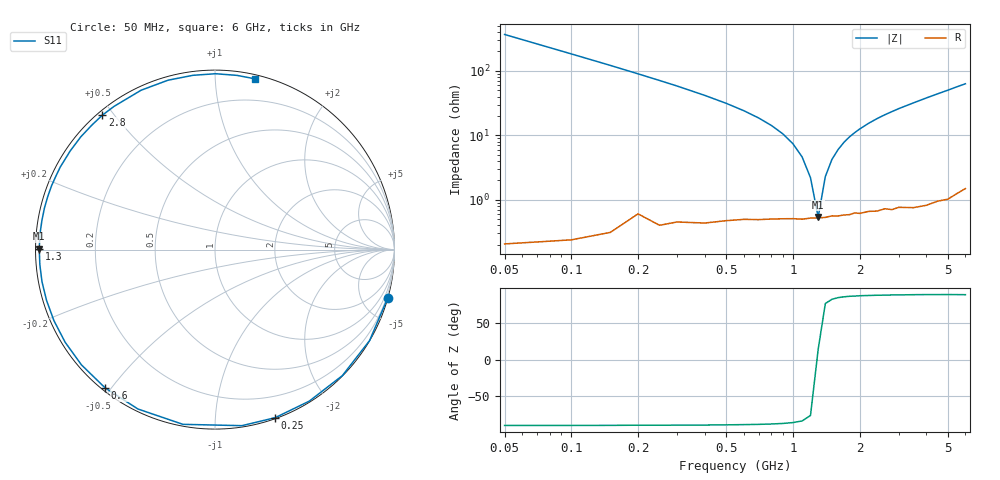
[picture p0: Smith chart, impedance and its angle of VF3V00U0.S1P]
! Infineon Technologies  Discrete & RF Semiconductors
! BBY 58-03
! Si Tuning Diode in SOD323
! VR = 3 V
! S-Parameters:  June  1999
# GHz  S  MA  R  50
!  f  S11
! GHz  MAG  ANG
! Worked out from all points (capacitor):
!   34 points, 50 MHz to 6 GHz, reference 50 ohm
!   read as one part to ground: C = 8.63 pF near 50 MHz
!   lowest |Z| = 539 mohm at 1.3 GHz (marker M1)
!   series resonance near 1.294 GHz, so ESL is about 1.8 nH
!   S11 on the Smith chart (normalised r, x): 50 MHz: 0.00, -7.35; 250 MHz: 0.01, -1.42; 600 MHz: 0.01, -0.48; 1.3 GHz: 0.01, +0.00; 2.8 GHz: 0.01, +0.47; 6 GHz: 0.03, +1.26
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0.05  0.9999 -15.5
0.1  0.9993 -30.5
0.15  0.9982 -44.7
0.2  0.9943 -58.1
0.25  0.9947 -70.3
0.3  0.9924 -81.3
0.4  0.9898 -100.4
0.5  0.9865 -115.8
0.6  0.984 -128.5
0.7  0.9829 -139.2
0.8  0.9816 -148.3
0.9  0.9808 -156.2
1  0.9803 -163.2
1.1  0.9804 -169.5
1.3  0.9793 179.7
1.5  0.9779 170.4
1.6  0.9781 166.3
1.8  0.9776 158.6
2  0.9772 151.9
2.4  0.9767 140.0
2.8  0.9772 129.9
3  0.9762 125.2
3.5  0.9788 114.9
4  0.9794 105.5
4.5  0.9788 97.2
5  0.9799 89.8
5.5  0.9784 82.8
6  0.9772 76.8
